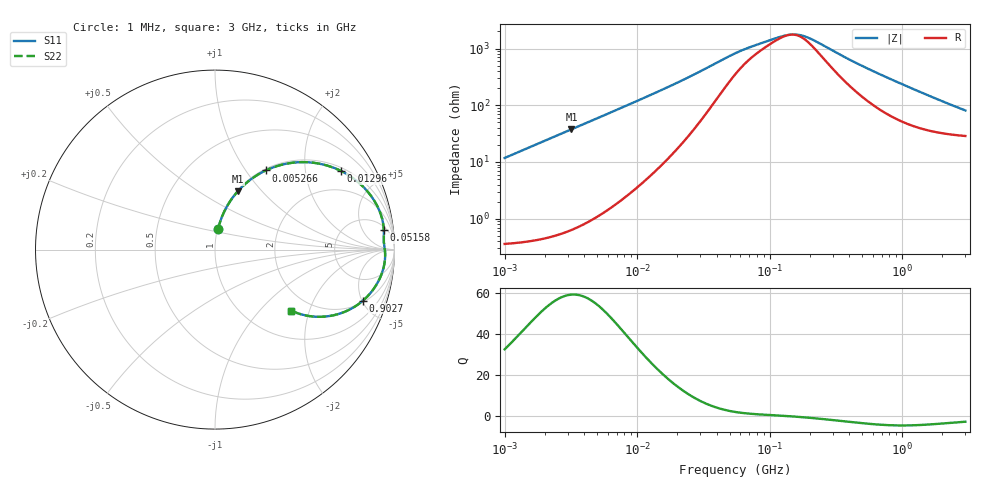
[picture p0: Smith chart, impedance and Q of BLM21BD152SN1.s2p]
! BLM21BD152SN1
# Hz S RI R 50
!Freq.(Hz) S11(Real) S11(Imag) S21(Real) S21(Imag) S12(Real) S12(Imag) S22(Real) S22(Imag)
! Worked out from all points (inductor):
!   401 points, 1 MHz to 3 GHz, reference 50 ohm
!   read as one part in series: L = 1.87 uH near 1.041 MHz
!   highest Q = 59.4 at 3.193 MHz (marker M1), where L = 1.87 uH
!   self-resonance near 144.2 MHz
!   S11 on the Smith chart (normalised r, x): 1 MHz: 1.01, +0.24; 5.266 MHz: 1.02, +1.24; 12.96 MHz: 1.12, +3.12; 51.58 MHz: 7, +14; 902.7 MHz: 2.15, -5.10; 3 GHz: 1.57, -1.51
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1000000  0.0171 0.1151  0.9829 -0.1151  0.9829 -0.1151  0.0171 0.1151
1935809  0.053 0.2146  0.947 -0.2146  0.947 -0.2146  0.053 0.2146
3192880  0.1279 0.3257  0.8721 -0.3257  0.8721 -0.3257  0.1279 0.3257
3823119  0.1728 0.3697  0.8272 -0.3697  0.8272 -0.3697  0.1728 0.3697
5266264  0.2823 0.4409  0.7177 -0.4409  0.7177 -0.4409  0.2823 0.4409
8345207  0.4956 0.4875  0.5044 -0.4875  0.5044 -0.4875  0.4956 0.4875
1.29622e7  0.7019 0.4384  0.2981 -0.4384  0.2981 -0.4384  0.7019 0.4384
1.461624e7  0.7488 0.4119  0.2512 -0.4119  0.2512 -0.4119  0.7488 0.4119
1.934349e7  0.8362 0.3391  0.1638 -0.3391  0.1638 -0.3391  0.8362 0.3391
2.611722e7  0.8965 0.257  0.1035 -0.257  0.1035 -0.257  0.8965 0.257
5.15801e7  0.9405 0.108  0.0595 -0.108  0.0595 -0.108  0.9405 0.108
5.477226e7  0.9407 0.0987  0.0593 -0.0987  0.0593 -0.0987  0.9407 0.0987
7.852918e7  0.94 0.0557  0.06 -0.0557  0.06 -0.0557  0.94 0.0557
1.348146e8  0.9454 0.0065  0.0546 -0.0065  0.0546 -0.0065  0.9454 0.0065
1.680187e8  0.9476 -0.0156  0.0524 0.0156  0.0524 0.0156  0.9476 -0.0156
2.094008e8  0.9479 -0.0401  0.0521 0.0401  0.0521 0.0401  0.9479 -0.0401
4.304467e8  0.926 -0.1418  0.074 0.1418  0.074 0.1418  0.926 -0.1418
8.005644e8  0.8498 -0.2601  0.1502 0.2601  0.1502 0.2601  0.8498 -0.2601
9.0272e8  0.8245 -0.2841  0.1755 0.2841  0.1755 0.2841  0.8245 -0.2841
1.67892e9  0.6313 -0.371  0.3687 0.371  0.3687 0.371  0.6313 -0.371
2.221924e9  0.5258 -0.3704  0.4742 0.3704  0.4742 0.3704  0.5258 -0.3704
3e9  0.4227 -0.3394  0.5773 0.3394  0.5773 0.3394  0.4227 -0.3394
